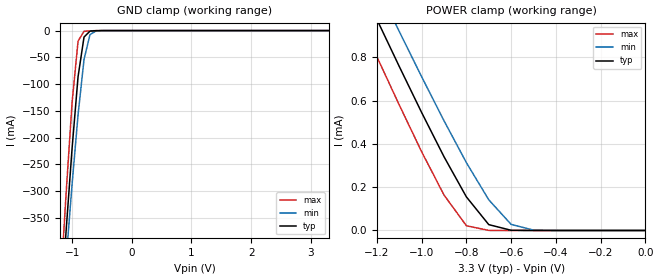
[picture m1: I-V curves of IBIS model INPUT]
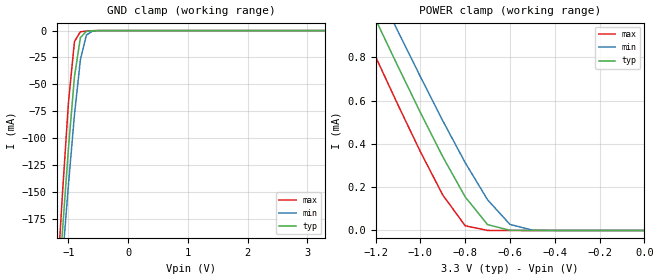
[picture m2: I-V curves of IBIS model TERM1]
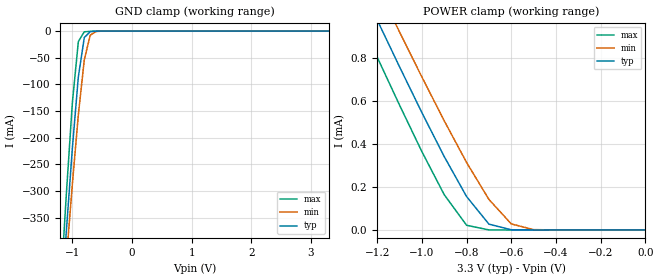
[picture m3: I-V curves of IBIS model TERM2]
|   PERICOM SEMICONDUCTOR CORP
|   IBIS Model of PI4MSD5V9546A
|   Product Family: 4MSD
|   SOIC-16 (W) Package
[IBIS Ver] 3.2
[Comment char] |_char
[File Name] pi4msd5v9546a_w_33v.ibs
[File Rev] 1.0
[Source] File originated at Pericom Semiconductor Corp.
[Date] 09/07/17
[Disclaimer] (C) Copyright PERICOM Semiconductor Corporation
   All rights reserved
  Pericom Semiconductor Corporation hereby grants the user of
  this IBIS model a non-exclusive, nontransferable license to
  use this IBIS model under the following terms.
  This IBIS model is provided on an "AS IS" basis and Pericom
  makes absolutely no warranty with respect to the information
  contained herein. PERICOM DISCLAIMS AND CUSTOMER WAIVES ALL
  WARRANTIES, EXPRESSED OR IMPLIED, INCLUDING WARRANTIES OF
  MERCHANTABILITY OR FITNESS FOR A PARTICULAR PURPOSE. The
  entire risk as to quality and performance is with the customer.
  Accordingly, in no event shall the company be liable for any
  damages, whether in contract or tort, including any lost
  profits or other incidental, consequential, exemplary, or
  punitive damages arising out of the use or application of the
  IBIS model provided in this package. Further, Pericom reserves
  the right to make changes without notice to any product herein
  to improve reliability, function, or design. Pericom does not
  convey any license under patent rights or any other intellectual
  property rights, including those of third parties.
  The user is granted this license only to use the IBIS model
  and is not granted rights to sell, load, rent, lease or license
  the IBIS model in whole or in part, or in modified form to anyone
  other than user. User may modify the IBIS model to suit its specific
  application but rights to derivative works and such modifications
  shall belong to Pericom.
  Pericom is not obligated to provide maintenance or support
  for the licensed IBIS model.
  Contact Pericom at ATTN: APPLICATION ENGINEERING / IBIS MODELS
  2380 Bering Drive, San Jose, CA 95131
[Component] PI4MSD5V9546A
[Manufacturer] Pericom Semiconductor Corp.
[Package]
| variable   typ   min   max
R_pkg   0.05665ohm   0.05334ohm   0.05997ohm
L_pkg   1.99150nH   1.82200nH   2.76100nH
C_pkg   0.20800pF   0.16300pF   0.25300pF
[Pin] signal_name   model_name   R_pin   L_pin   C_pin
1   A0   INPUT   0.05997   2.76100nH   0.25300pF
2   A1   INPUT   0.05776   2.54800nH   0.22300pF
3   _RESET   INPUT   0.05555   2.33500nH   0.19300pF
4   SD0   TERM1   0.05334   2.12200nH   0.16300pF
5   SC0   TERM1   0.05334   2.12200nH   0.16300pF
6   SD1   TERM1   0.05555   2.33500nH   0.19300pF
7   SC1   TERM1   0.05776   2.54800nH   0.22300pF
8   GND   GND   0.05997   2.76100nH   0.25300pF
9   SD2   TERM1   0.05997   2.76100nH   0.25300pF
10   SC2   TERM1   0.05776   2.54800nH   0.22300pF
11   SD3   TERM1   0.05555   2.33500nH   0.19300pF
12   SC3   TERM1   0.05334   2.12200nH   0.16300pF
13   A2   INPUT   0.05334   2.12200nH   0.16300pF
14   SCL   TERM2   0.05555   2.33500nH   0.19300pF
15   SDA   TERM2   0.05776   2.54800nH   0.22300pF
16   VCC   POWER   0.05997   2.76100nH   0.25300pF
[Series Switch Groups]
On 1 /
Off 2 3 4 /
[Series Pin Mapping]   pin_2   model_name  function_table_group
4   15   SWITCH1   1
5   14   SWITCH1   1
6   15   SWITCH1   2
7   14   SWITCH1   2
9   15   SWITCH1   3
10   14   SWITCH1   3
11   15   SWITCH1   4
12   14   SWITCH1   4
|   Model SWITCH1
[Model] SWITCH1
Model_type Series_switch
| variable   typ   min   max
C_comp   6.96pF   6.94pF   6.98pF
[Voltage Range]   3.3000V   3.0000V   3.6000V
[GND Clamp Reference]   0.0000V   0.0000V   0.0000V
[POWER Clamp Reference]   3.3000V   3.0000V   3.6000V
[Temperature Range]   25   85   -40
[On]
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[OFF]
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| Models and submodels in the file (4): INPUT (Input), SWITCH1 (Series_switch), TERM1 (Terminator), TERM2 (Terminator)
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|   Model INPUT
[Model] INPUT
Model_type Input
Vinl = 990mV
Vinh = 2.31V
| variable   typ   min   max
C_comp   4.38pF   4.37pF   4.39pF
[Voltage Range]   3.3000V   3.0000V   3.6000V
[GND Clamp Reference]   0.0000V   0.0000V   0.0000V
[POWER Clamp Reference]   3.3000V   3.0000V   3.6000V
[Temperature Range]   25   85   -40
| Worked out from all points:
|   GND clamp passes 1 mA (typ) near -0.70 V on its own axis
|   POWER clamp passes 1 mA (typ) near -1.21 V on its own axis
[GND Clamp]
| Voltage   I(typ)   I(min)   I(max)
-3.3V     -4.214A    -3.861A    -4.708A
-1.2V     -536.3mA   -573.9mA   -488.8mA
-1.1V     -373.8mA   -427.8mA   -304mA
-1V       -219.8mA   -287.2mA   -134.4mA
-900mV    -86.22mA   -157.4mA   -19.74mA
-800mV    -12.06mA   -53.77mA   -1.311mA
-700mV    -1.032mA   -7.522mA   -526.9uA
-600mV    -210.6uA   -734.5uA   -129.9uA
3.3V      125.8pA    2.663nA    123.3pA
[POWER Clamp]   |Note: Vtable = Vcc - Voutput
| Voltage   I(typ)   I(min)   I(max)
-3.3V     5.749mA    5.788mA    5.712mA
-1.3V     1.195mA    1.347mA    1.029mA
-1.2V     974.9uA    1.132mA    802.5uA
-1.1V     757.6uA    919.3uA    579.7uA
-1V       544.9uA    710.2uA    363.8uA
-900mV    340.5uA    506.6uA    163.7uA
-800mV    155.1uA    313.2uA    21.83uA
-700mV    27.01uA    141.6uA    235.8nA
-600mV    852.5nA    28.01uA    1.791nA
-500mV    17.74nA    1.596uA    170.4pA
0V        125.8pA    153.2pA    136.8pA
|   Model TERM1
[Model] TERM1
Model_type Terminator
| variable   typ   min   max
C_comp   2.58pF   2.57pF   2.59pF
[Voltage Range]   3.3000V   3.0000V   3.6000V
[GND Clamp Reference]   0.0000V   0.0000V   0.0000V
[POWER Clamp Reference]   3.3000V   3.0000V   3.6000V
[Temperature Range]   25   85   -40
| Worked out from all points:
|   GND clamp passes 1 mA (typ) near -0.70 V on its own axis
|   POWER clamp passes 1 mA (typ) near -1.21 V on its own axis
[GND Clamp]
| Voltage   I(typ)   I(min)   I(max)
-3.3V     -2.1A      -1.924A    -2.346A
-1.2V     -267.2mA   -286mA     -243.4mA
-1.1V     -186.2mA   -213.2mA   -151.2mA
-1V       -109.4mA   -143.1mA   -66.79mA
-900mV    -42.98mA   -78.43mA   -10.22mA
-800mV    -6.45mA    -26.94mA   -1.105mA
-700mV    -805uA     -4.15mA    -477.3uA
-600mV    -185.9uA   -544.9uA   -115.7uA
3.3V      68.73pA    2.569nA    67.15pA
[POWER Clamp]   |Note: Vtable = Vcc - Voutput
| Voltage   I(typ)   I(min)   I(max)
-3.3V     5.749mA    5.788mA    5.712mA
-1.3V     1.195mA    1.347mA    1.029mA
-1.2V     974.9uA    1.132mA    802.5uA
-1.1V     757.6uA    919.3uA    579.7uA
-1V       544.9uA    710.2uA    363.8uA
-900mV    340.5uA    506.6uA    163.7uA
-800mV    155.1uA    313.2uA    21.83uA
-700mV    27.01uA    141.6uA    235.7nA
-600mV    852.4nA    28.01uA    1.717nA
-500mV    17.67nA    1.596uA    99.08pA
0V        68.73pA    67.71pA    74.93pA
|   Model TERM2
[Model] TERM2
Model_type Terminator
| variable   typ   min   max
C_comp   4.38pF   4.37pF   4.39pF
[Voltage Range]   3.3000V   3.0000V   3.6000V
[GND Clamp Reference]   0.0000V   0.0000V   0.0000V
[POWER Clamp Reference]   3.3000V   3.0000V   3.6000V
[Temperature Range]   25   85   -40
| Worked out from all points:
|   GND clamp passes 1 mA (typ) near -0.70 V on its own axis
|   POWER clamp passes 1 mA (typ) near -1.21 V on its own axis
[GND Clamp]
| Voltage   I(typ)   I(min)   I(max)
-3.3V     -4.214A    -3.861A    -4.708A
-1.2V     -536.3mA   -573.9mA   -488.8mA
-1.1V     -373.8mA   -427.8mA   -304mA
-1V       -219.8mA   -287.2mA   -134.4mA
-900mV    -86.22mA   -157.4mA   -19.74mA
-800mV    -12.06mA   -53.77mA   -1.311mA
-700mV    -1.032mA   -7.522mA   -526.9uA
-600mV    -210.6uA   -734.5uA   -129.9uA
3.3V      125.8pA    2.663nA    123.3pA
[POWER Clamp]   |Note: Vtable = Vcc - Voutput
| Voltage   I(typ)   I(min)   I(max)
-3.3V     5.749mA    5.788mA    5.712mA
-1.3V     1.195mA    1.347mA    1.029mA
-1.2V     974.9uA    1.132mA    802.5uA
-1.1V     757.6uA    919.3uA    579.7uA
-1V       544.9uA    710.2uA    363.8uA
-900mV    340.5uA    506.6uA    163.7uA
-800mV    155.1uA    313.2uA    21.83uA
-700mV    27.01uA    141.6uA    235.8nA
-600mV    852.5nA    28.01uA    1.791nA
-500mV    17.74nA    1.596uA    170.4pA
0V        125.8pA    153.2pA    136.8pA
